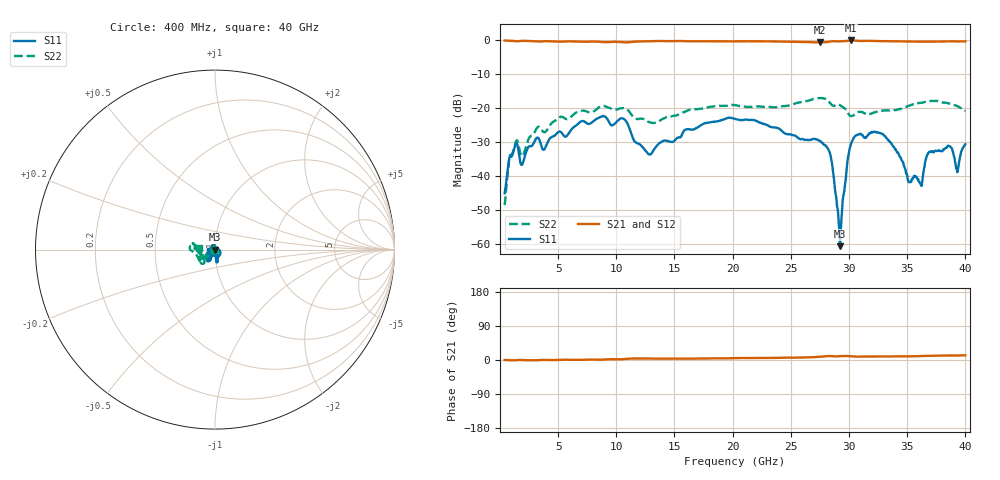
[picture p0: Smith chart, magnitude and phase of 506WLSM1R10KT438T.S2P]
!  American Technical Ceramics  Date:  8/31/2012
!  One Norden Lane
!  Huntington Station,  NY.  11746-2102
!  Tel:  (631) 622-4700  Fax:  (631) 622-4748
!  Part Number  506WLSM1R10KT438T
!  Description:  Ultra-Broadband Inductor
!  Application:  Ultra-broadband DC block decoupling, bias tee
# GHZ S DB R 50
! Freq  |S11|  S11 Ph  |S21|  S21 Ph  |S12|  S12 Ph  |S22|  S22 Ph
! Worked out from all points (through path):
!   801 points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, 400 MHz to 40 GHz, reference 50 ohm
!   highest |S21| = -0.01 dB at 30.15 GHz (marker M1); lowest = -0.6 dB at 27.48 GHz (marker M2)
!   lowest |S11| = -60.7 dB at 29.21 GHz (marker M3), VSWR 1.00, Z = 49.9 - j0.00506 ohm
!   |S11| at or under -10 dB: start of sweep to end of sweep
!   |S22| runs from -48.5 to -17.0 dB; largest |S21 - S12| = 0.0024
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0.4  -45.06 178.9  -0.03 0.1  -0.03 0.1  -48.55 179.0
0.8455  -34.09 -142.1  -0.12 -0.7  -0.12 -0.7  -33.88 -128.4
1.39  -30.40 -159.2  -0.24 -0.6  -0.24 -0.6  -29.64 -147.3
1.9345  -36.43 -150.0  -0.12 -0.1  -0.12 -0.1  -34.10 -148.6
3.2215  -28.66 -149.0  -0.32 -0.5  -0.32 -0.5  -25.66 -143.7
7.033  -23.77 -118.9  -0.39 0.4  -0.39 0.5  -20.74 -136.4
10.5475  -22.99 -132.7  -0.53 2.2  -0.52 2.2  -19.95 -143.6
12.7255  -33.38 -116.1  -0.24 4.0  -0.23 4.0  -23.94 -154.8
13.6165  -30.57 -89.0  -0.17 3.5  -0.16 3.5  -23.91 -146.2
20.2  -23.10 -82.8  -0.29 4.9  -0.28 4.9  -19.10 -142.7
26.833  -29.12 -106.7  -0.53 7.3  -0.52 7.3  -17.41 -178.1
27.4765  -29.57 -147.9  -0.59 8.5  -0.57 8.5  -16.98 177.1
28.3675  -33.44 124.9  -0.34 10.5  -0.33 10.5  -18.45 168.7
29.209  -60.65 -176.9  -0.28 10.2  -0.27 10.2  -19.04 174.6
30.1495  -30.78 -16.2  -0.01 9.9  -0.01 9.9  -22.29 -176.1
33.4165  -29.61 -76.6  -0.24 9.4  -0.25 9.4  -20.62 -167.1
35.149  -41.83 -25.9  -0.32 9.6  -0.31 9.6  -19.24 175.4
36.0895  -41.99 48.1  -0.40 10.4  -0.40 10.4  -18.43 166.4
36.931  -32.82 93.6  -0.35 11.0  -0.36 11.0  -17.86 164.4
38.6635  -31.19 118.8  -0.28 11.9  -0.28 11.9  -18.66 167.2
39.307  -38.87 154.6  -0.30 11.8  -0.28 11.8  -19.37 169.2
40  -30.59 -164.8  -0.28 12.2  -0.27 12.2  -20.81 174.4
